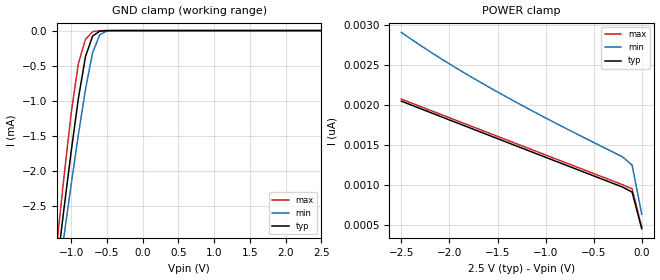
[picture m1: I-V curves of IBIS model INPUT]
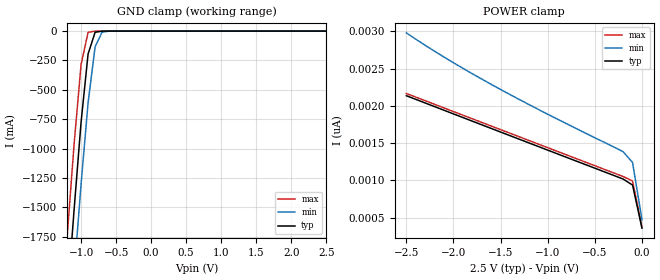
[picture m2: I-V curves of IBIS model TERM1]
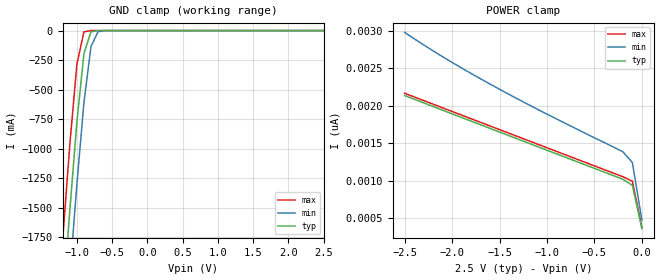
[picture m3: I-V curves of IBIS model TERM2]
|   PERICOM SEMICONDUCTOR CORP
|   IBIS Model of PI3CH360
|   Product Family: 3CH
|   TSSOP (L) Package
[IBIS Ver] 3.2
[Comment char] |_char
[File Name] pi3ch360_l_25v.ibs
[File Rev] 1.0
[Source] File originated at Pericom Semiconductor Corp.
[Date] 3/18/15
[Disclaimer] (C) Copyright PERICOM Semiconductor Corporation
   All rights reserved
  Pericom Semiconductor Corporation hereby grants the user of
  this IBIS model a non-exclusive, nontransferable license to
  use this IBIS model under the following terms.
  This IBIS model is provided on an "AS IS" basis and Pericom
  makes absolutely no warranty with respect to the information
  contained herein. PERICOM DISCLAIMS AND CUSTOMER WAIVES ALL
  WARRANTIES, EXPRESSED OR IMPLIED, INCLUDING WARRANTIES OF
  MERCHANTABILITY OR FITNESS FOR A PARTICULAR PURPOSE. The
  entire risk as to quality and performance is with the customer.
  Accordingly, in no event shall the company be liable for any
  damages, whether in contract or tort, including any lost
  profits or other incidental, consequential, exemplary, or
  punitive damages arising out of the use or application of the
  IBIS model provided in this package. Further, Pericom reserves
  the right to make changes without notice to any product herein
  to improve reliability, function, or design. Pericom does not
  convey any license under patent rights or any other intellectual
  property rights, including those of third parties.
  The user is granted this license only to use the IBIS model
  and is not granted rights to sell, load, rent, lease or license
  the IBIS model in whole or in part, or in modified form to anyone
  other than user. User may modify the IBIS model to suit its specific
  application but rights to derivative works and such modifications
  shall belong to Pericom.
  Pericom is not obligated to provide maintenance or support
  for the licensed IBIS model.
  Contact Pericom at ATTN: APPLICATION ENGINEERING / IBIS MODELS
  3545 North First Street, San Jose, CA 95134
[Component] PI3CH360
[Manufacturer] Pericom Semiconductor Corp.
[Package]
| variable   typ   min   max
R_pkg   0.05666ohm   0.05334ohm   0.05997ohm
L_pkg   2.99150nH   2.22200nH   3.76100nH
C_pkg   0.20800pF   0.16300pF   0.25300pF
[Pin]  signal_name   model_name   R_pin   L_pin   C_pin
1   S   INPUT   0.05997   3.76100nH   0.25300pF
2   NC   NC   0.05776   3.24800nH   0.22300pF
3   NC   NC   0.05555   2.73500nH   0.19300pF
4   YA   TERM2   0.05334   2.22200nH   0.16300pF
5   YB   TERM2   0.05334   2.22200nH   0.16300pF
6   YC   TERM2   0.05555   2.73500nH   0.19300pF
7   NC   NC   0.05776   3.24800nH   0.22300pF
8   GND   GND   0.05997   3.76100nH   0.25300pF
9   IC1   TERM1   0.05997   3.76100nH   0.25300pF
10   IB1   TERM1   0.05776   3.24800nH   0.22300pF
11   IA1   TERM1   0.05555   2.73500nH   0.19300pF
12   IC0   TERM1   0.05334   2.22200nH   0.16300pF
13   IB0   TERM1   0.05334   2.22200nH   0.16300pF
14   IA0   TERM1   0.05555   2.73500nH   0.19300pF
15   /EN   INPUT   0.05776   3.24800nH   0.22300pF
16   VCC   POWER   0.05997   3.76100nH   0.25300pF
[Series Switch Groups]
On 1 /
Off 2 /
[Series Pin Mapping]   pin_2   model_name  function_table_group
14   4   SWITCH1   1
13   5   SWITCH1   1
12   6   SWITCH1   1
11   4   SWITCH1   2
10   5   SWITCH1   2
9   6   SWITCH1   2
|   Model SWITCH1
[Model] SWITCH1
Model_type Series_switch
| variable   typ   min   max
C_comp   6.40pF   6.30pF   6.50pF
[Voltage Range]   2.500V   2.250V   2.750V
[GND Clamp Reference]   0.000V   0.000V   0.000V
[POWER Clamp Reference]   2.500V   2.250V   2.750V
[On]
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[OFF]
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| Models and submodels in the file (4): INPUT (Input), SWITCH1 (Series_switch), TERM1 (Terminator), TERM2 (Terminator)
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|   Model INPUT
[Model] INPUT
Model_type Input
Vinl = 0.800V
Vinh = 1.800V
| variable   typ   min   max
C_comp   1.800pF   1.700pF   1.900pF
[Voltage Range]   2.500V   2.250V   2.750V
[GND Clamp Reference]   0.000V   0.000V   0.000V
[POWER Clamp Reference]   2.500V   2.250V   2.750V
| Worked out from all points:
|   GND clamp passes 1 mA (typ) near -0.90 V on its own axis
[GND Clamp]
| Voltage   I(typ)   I(min)  I(max)
-2.5V     -14.74mA   -13.73mA   -16.44mA
-1.2V     -3.364mA   -3.668mA   -3.042mA
-1.1V     -2.528mA   -2.921mA   -2.075mA
-1V       -1.72mA    -2.189mA   -1.175mA
-900mV    -970.6uA   -1.485mA   -470.9uA
-800mV    -370.2uA   -835.9uA   -124.8uA
-700mV    -77.27uA   -313.6uA   -15.69uA
-600mV    -8.132uA   -56.97uA   -899.1nA
-500mV    -581.9nA   -5.514uA   -27.41nA
2.5V      456.5pA    1.382nA    21.38pA
[POWER Clamp]   |Note: Vtable = Vcc - Voutput
| Voltage   I(typ)   I(min)   I(max)
-2.5V     2.046nA    2.904nA    2.072nA
-2.1V     1.859nA    2.586nA    1.886nA
-1.6V     1.626nA    2.228nA    1.654nA
-1V       1.347nA    1.838nA    1.376nA
-200mV    975.5pA    1.351nA    1.005nA
-100mV    912.5pA    1.249nA    952.9pA
0V        456.5pA    636.6pA    471.6pA
|   Model TERM1
[Model] TERM1
Model_type Terminator
| variable   typ   min   max
C_comp   3.200pF   3.150pF   3.350pF
[Voltage Range]   2.500V   2.250V   2.750V
[GND Clamp Reference]   0.000V   0.000V   0.000V
[POWER Clamp Reference]   2.500V   2.250V   2.750V
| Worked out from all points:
|   GND clamp passes 1 mA (typ) near -0.71 V on its own axis
[GND Clamp]
| Voltage   I(typ)   I(min)   I(max)
-2.5V     -12.6A     -12.86A    -12.34A
-1.2V     -2.312A    -2.839A    -1.76A
-1.1V     -1.522A    -2.068A    -964.6mA
-1V       -774.2mA   -1.302A    -284.3mA
-900mV    -194.8mA   -609.8mA   -10.79mA
-800mV    -10.29mA   -134.3mA   -176uA
-700mV    -369.5uA   -9.267mA   -1.644uA
-500mV    -244.1nA   -27.85uA   -129.7pA
2.5V      361.1pA    1.419nA    73.2pA
[POWER Clamp]   |Note: Vtable = Vcc - Voutput
| Voltage   I(typ)   I(min)   I(max)
-2.5V     2.136nA    2.978nA    2.166nA
-2.1V     1.941nA    2.654nA    1.972nA
-1.6V     1.698nA    2.289nA    1.73nA
-1V       1.407nA    1.888nA    1.44nA
-200mV    1.019nA    1.386nA    1.053nA
-100mV    938.7pA    1.242nA    993.5pA
0V        361.1pA    474.5pA    376.7pA
|   Model TERM2
[Model] TERM2
Model_type Terminator
| variable   typ   min   max
C_comp   3.200pF   3.150pF   3.350pF
[Voltage Range]   2.500V   2.250V   2.750V
[GND Clamp Reference]   0.000V   0.000V   0.000V
[POWER Clamp Reference]   2.500V   2.250V   2.750V
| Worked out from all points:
|   GND clamp passes 1 mA (typ) near -0.71 V on its own axis
[GND Clamp]
| Voltage   I(typ)   I(min)   I(max)
-2.5V     -12.6A     -12.86A    -12.34A
-1.2V     -2.312A    -2.839A    -1.76A
-1.1V     -1.522A    -2.068A    -964.6mA
-1V       -774.2mA   -1.302A    -284.3mA
-900mV    -194.8mA   -609.8mA   -10.79mA
-800mV    -10.29mA   -134.3mA   -176uA
-700mV    -369.5uA   -9.267mA   -1.644uA
-500mV    -244.1nA   -27.85uA   -129.7pA
2.5V      361.1pA    1.419nA    73.2pA
[POWER Clamp]   |Note: Vtable = Vcc - Voutput
| Voltage   I(typ)   I(min)   I(max)
-2.5V     2.136nA    2.978nA    2.166nA
-2.1V     1.941nA    2.654nA    1.972nA
-1.6V     1.698nA    2.289nA    1.73nA
-1V       1.407nA    1.888nA    1.44nA
-200mV    1.019nA    1.386nA    1.053nA
-100mV    938.7pA    1.242nA    993.5pA
0V        361.1pA    474.6pA    376.7pA
